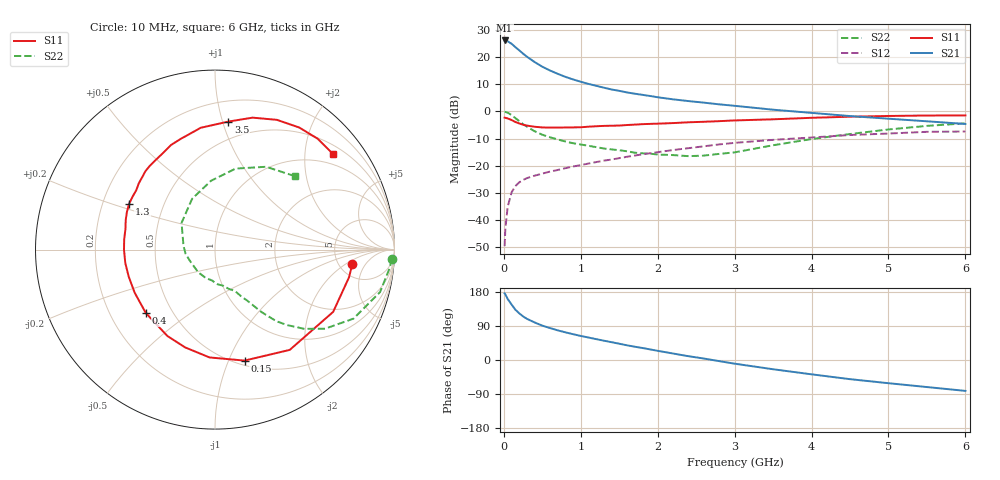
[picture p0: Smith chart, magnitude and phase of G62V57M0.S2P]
! SIEMENS Small Signal Semiconductors
! BFG193
! Si NPN RF Bipolar Junction Transistor in SOT223
! VCE = 2.5 V  IC = 7 mA
! Common Emitter S-Parameters:  August  1996
# GHz  S  MA  R  50
!  f  S11  S21  S12  S22
! GHz  MAG  ANG  MAG  ANG  MAG  ANG  MAG  ANG
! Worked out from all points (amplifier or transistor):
!   36 points, 10 MHz to 6 GHz, reference 50 ohm
!   highest |S21| = 26.2 dB at 10 MHz (marker M1)
!   |S21| within 3 dB of that: start of sweep to 173 MHz
!   unconditionally stable (mu >= 1): 969.3 MHz to 2.627 GHz
!   at 250 MHz: K = 0.43, MSG = 23.3 dB, |S12| = -25.2 dB
!   at 1.4 GHz: K = 1.08, MAG = 11.2 dB, |S12| = -17.7 dB
!   at 6 GHz: K = 0.89, MSG = 1.4 dB, |S12| = -7.4 dB
!   S11 on the Smith chart (normalised r, x): 10 MHz: 6.69, -2.55; 150 MHz: 0.55, -1.14; 400 MHz: 0.36, -0.35; 1.3 GHz: 0.31, +0.23; 3.5 GHz: 0.36, +1.05; 6 GHz: 0.71, +2.65
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0.01  0.7697 -5.8  20.34 175.9  0.0033 92.0  0.9859 -3.0
0.02  0.7625 -11.7  20.31 173.0  0.007 87.6  0.9792 -5.9
0.05  0.7442 -27.8  19.62 161.0  0.0175 76.0  0.9497 -14.4
0.1  0.6969 -53.3  17.69 146.5  0.0322 65.9  0.862 -26.5
0.15  0.6399 -75.1  15.32 132.7  0.0422 57.2  0.7552 -35.7
0.2  0.6016 -92.9  13.38 123.2  0.0495 52.0  0.665 -41.6
0.25  0.5698 -107.0  11.62 115.0  0.0547 48.3  0.5831 -46.2
0.3  0.5495 -118.9  10.21 108.7  0.0592 46.1  0.5259 -49.4
0.4  0.5227 -137.5  8.141 99.1  0.0657 43.9  0.4322 -53.4
0.5  0.508 -151.8  6.676 90.7  0.0716 42.8  0.373 -55.8
0.6  0.5038 -162.6  5.687 84.3  0.0781 43.0  0.3348 -57.8
0.7  0.5054 -171.5  4.94 78.3  0.0835 43.0  0.3053 -60.2
0.9  0.5092 173.5  3.891 68.1  0.0969 43.2  0.26 -63.9
1.1  0.5243 161.5  3.22 59.3  0.1098 43.3  0.2331 -70.4
1.3  0.5424 151.9  2.744 51.0  0.1241 42.2  0.208 -76.6
1.7  0.5722 135.1  2.127 35.1  0.1539 38.6  0.174 -94.6
2.2  0.6111 118.3  1.673 17.1  0.1948 31.3  0.1572 -126.3
2.8  0.6631 101.4  1.353 -3.0  0.2473 20.6  0.1655 -172.1
3.5  0.7173 84.0  1.078 -24.4  0.3001 5.0  0.2385 141.4
4.5  0.801 64.5  0.823 -50.6  0.3686 -15.0  0.3842 93.3
5.5  0.8419 47.2  0.659 -71.4  0.4216 -39.5  0.5424 58.3
6  0.846 39.1  0.589 -81.5  0.4273 -53.6  0.6052 42.5
